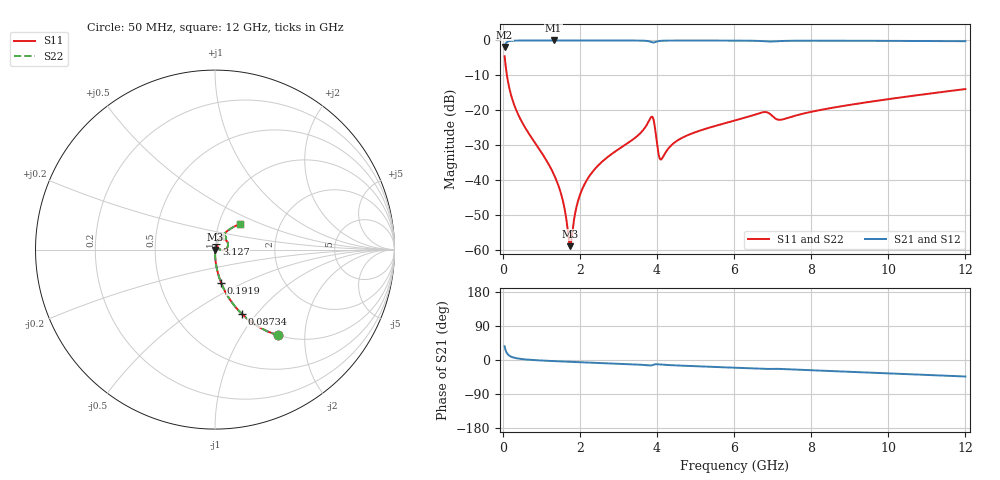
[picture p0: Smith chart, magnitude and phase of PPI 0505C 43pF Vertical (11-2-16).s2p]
# GHz S MA R 50
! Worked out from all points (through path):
!   1601 points, 50 MHz to 12 GHz, reference 50 ohm
!   highest |S21| = -0.01 dB at 1.32 GHz (marker M1); lowest = -1.9 dB at 50 MHz (marker M2)
!   group delay of S21, straight-line fit = 10.8 ps
!   lowest |S11| = -58.9 dB at 1.745 GHz (marker M3), VSWR 1.00, Z = 50.1 - j0.0199 ohm
!   |S11| at or under -10 dB: 110.3 MHz to end of sweep
!   |S22| runs from -58.9 to -4.5 dB; largest |S21 - S12| = 0
!   S11 on the Smith chart (normalised r, x): 50 MHz: 1.00, -1.47; 87.34 MHz: 1.00, -0.84; 191.9 MHz: 1.00, -0.38; 3.127 GHz: 1.01, +0.06; 12 GHz: 1.27, +0.38
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0.05  0.5936 -53.7  0.8045 36.3  0.8045 36.3  0.5936 -53.7
0.08734375  0.3884 -67.3  0.9212 22.6  0.9212 22.6  0.3884 -67.3
0.1919063  0.1867 -79.6  0.982 10.2  0.982 10.2  0.1867 -79.6
0.4757188  0.0718 -86.7  0.9968 2.8  0.9968 2.8  0.0718 -86.7
1.319687  0.0123 -88.3  0.9989 -2.9  0.9989 -2.9  0.0123 -88.3
1.54375  0.005529 -82.8  0.9988 -3.9  0.9988 -3.9  0.005529 -82.8
1.745406  0.001132 -10.1  0.9988 -4.8  0.9988 -4.8  0.001132 -10.1
1.924656  0.00436 68.7  0.9987 -5.5  0.9987 -5.5  0.00436 68.7
2.044156  0.007014 74.0  0.9986 -6.0  0.9986 -6.0  0.007014 74.0
2.432531  0.01529 77.3  0.9984 -7.5  0.9984 -7.5  0.01529 77.3
3.127125  0.03068 76.1  0.9974 -10.3  0.9974 -10.3  0.03068 76.1
3.859062  0.08057 37.8  0.9481 -14.2  0.9481 -14.2  0.08057 37.8
3.926281  0.06755 8.0  0.936 -12.0  0.936 -12.0  0.06755 8.0
4.038312  0.02427 6.2  0.9766 -11.4  0.9766 -11.4  0.02427 6.2
4.120469  0.01998 40.2  0.9874 -12.1  0.9874 -12.1  0.01998 40.2
4.665687  0.04063 70.6  0.9958 -15.0  0.9958 -15.0  0.04063 70.6
6.025  0.07128 66.7  0.9935 -20.4  0.9935 -20.4  0.07128 66.7
6.764406  0.094 54.6  0.976 -23.6  0.976 -23.6  0.094 54.6
7.190125  0.07295 52.0  0.9787 -23.5  0.9787 -23.5  0.07295 52.0
8.019156  0.09546 60.1  0.9903 -27.1  0.9903 -27.1  0.09546 60.1
10.01331  0.1445 53.5  0.9854 -35.2  0.9854 -35.2  0.1445 53.5
12  0.2011 45.4  0.975 -43.5  0.975 -43.5  0.2011 45.4
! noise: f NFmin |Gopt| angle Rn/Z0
0.05  0.0003713  0.8588  0.6293  0.0005628
1.372  0.003764  0.6581  3.809  0.0021
2.701  0.006508  0.6201  7.242  0.003183
4.031  0.03178  0.8665  10.98  0.05069
5.36  0.01222  0.6045  14.15  0.005626
6.682  0.03066  0.7824  17.94  0.02822
8.012  0.01955  0.628  21.01  0.00954
9.341  0.01853  0.5631  23.84  0.007331
10.67  0.02006  0.5468  26.76  0.007499
12  0.02215  0.5428  29.65  0.008092
